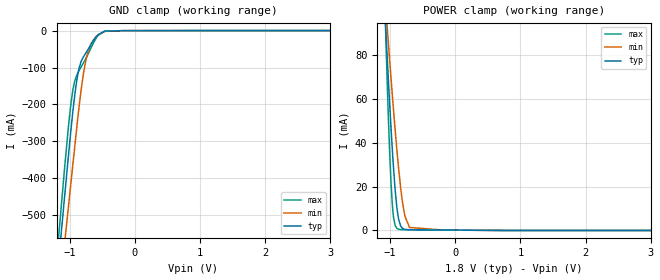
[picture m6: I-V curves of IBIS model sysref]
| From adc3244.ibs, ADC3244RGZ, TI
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|   sysref Model
[Model]   sysref
Model_type   Input
Vinl = 0.4
Vinh = 1.2
|   typ   min   max
|   (nom PVT)   (fast PVT)   (slow PVT)
C_comp   1.444e-12   1.378e-12   1.516e-12
| Where nom  PVT is Nominal Process, 1.8V, 27C
|   Fast PVT is Strong Process,  1.9V, -40C
|   Slow PVT is Weak Process,   1.7V, 125C
[Voltage Range]   1.8   1.7   1.9
|Junction Temperature
[Temperature Range]   27   125   -40
[Power Clamp Reference]   1.8   1.7   1.9
[GND Clamp Reference]   0   0   0
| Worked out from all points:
|   POWER clamp passes 1 mA (typ) near -0.81 V on its own axis
[GND Clamp]
|   Voltage   I(typ)   I(min)   I(max)
-1.8V     -1.831A    -1.819A    -1.858A
-1.364V   -995mA     -1.066A    -959.2mA
-1.076V   -449.2mA   -575.4mA   -371.3mA
-1.018V   -341mA     -478.1mA   -261.6mA
-956.4mV  -231.1mA   -374.9mA   -169.2mA
-864mV    -110.1mA   -222.3mA   -111.5mA
-811.8mV  -79.42mA   -147.3mA   -95.12mA
-747.7mV  -60.24mA   -78.64mA   -75.21mA
-662.7mV  -35.46mA   -33.28mA   -44mA
-560.7mV  -11.17mA   -11.17mA   -12.99mA
-180mV    -221.8uA   -172.1uA   -336.9uA
3.6V      0A         0A         0A
[POWER Clamp]
|   Voltage   I(typ)   I(min)   I(max)
-1.8V     579.9mA    428.1mA    963.1mA
-1.074V   95.85mA    104.5mA    95.3mA
-1.042V   76.85mA    91.26mA    64.08mA
-1.008V   57.75mA    77.59mA    35.51mA
-986.8mV  46.71mA    69.41mA    21.58mA
-948.6mV  28.5mA     54.94mA    6.124mA
-895.6mV  10.06mA    36.32mA    921.3uA
-873mV    5.512mA    29.11mA    566.5uA
-813.6mV  1.021mA    13.41mA    379.7uA
-774.9mV  489.5uA    6.65mA     361.6uA
-703.5mV  315.9uA    1.386mA    342.7uA
3.6V      0A         0A         0A
